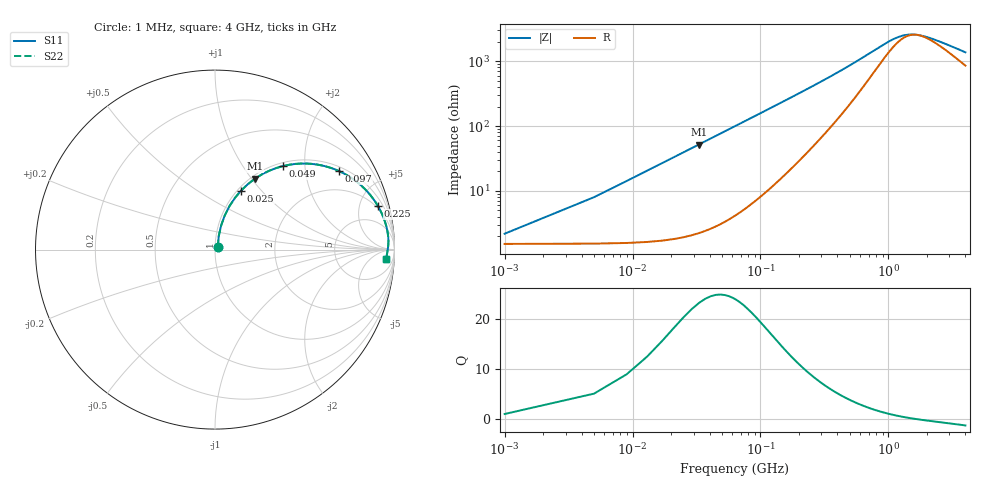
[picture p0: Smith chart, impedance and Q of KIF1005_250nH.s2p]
!version-2
!date-12.2020
!Series
# MHz S RI R 50
!Freq ReS11 ImS11 ReS21 ImS21 ReS12 ImS12 ReS22 ImS22
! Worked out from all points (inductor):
!   1001 points, 1 MHz to 4 GHz, reference 50 ohm
!   read as one part in series: L = 250 nH near 21 MHz
!   highest Q = 22.9 at 33 MHz (marker M1), where L = 250 nH
!   self-resonance near 1.67 GHz
!   S11 on the Smith chart (normalised r, x): 1 MHz: 1.03, +0.03; 25 MHz: 1.04, +0.79; 49 MHz: 1.06, +1.54; 97 MHz: 1.15, +3.06; 225 MHz: 1.73, +7.18; 4 GHz: 18, -21
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1  0.0152 0.0152  0.9848 -0.0152  0.9848 -0.0152  0.0152 0.0152
13  0.0542 0.1899  0.9458 -0.1899  0.9458 -0.1899  0.0542 0.1899
25  0.1457 0.3291  0.8543 -0.3291  0.8543 -0.3291  0.1457 0.3291
33  0.2218 0.3945  0.7782 -0.3945  0.7782 -0.3945  0.2218 0.3945
49  0.3773 0.4651  0.6227 -0.4651  0.6227 -0.4651  0.3773 0.4651
73  0.5662 0.4742  0.4338 -0.4742  0.4338 -0.4742  0.5662 0.4742
97  0.6917 0.4372  0.3083 -0.4372  0.3083 -0.4372  0.6917 0.4372
121  0.7721 0.3911  0.2279 -0.3911  0.2279 -0.3911  0.7721 0.3911
149  0.8315 0.3411  0.1685 -0.3411  0.1685 -0.3411  0.8315 0.3411
225  0.9074 0.2433  0.0926 -0.2433  0.0926 -0.2433  0.9074 0.2433
309  0.9385 0.1791  0.0615 -0.1791  0.0615 -0.1791  0.9385 0.1791
409  0.9539 0.1325  0.0461 -0.1325  0.0461 -0.1325  0.9539 0.1325
669  0.9651 0.0708  0.0349 -0.0708  0.0349 -0.0708  0.9651 0.0708
841  0.9662 0.0488  0.0338 -0.0488  0.0338 -0.0488  0.9662 0.0488
1009  0.9659 0.0338  0.0341 -0.0338  0.0341 -0.0338  0.9659 0.0338
1169  0.9652 0.0229  0.0348 -0.0229  0.0348 -0.0229  0.9652 0.0229
1337  0.9642 0.0137  0.0358 -0.0137  0.0358 -0.0137  0.9642 0.0137
1609  0.9626 0.00219  0.0374 -0.00219  0.0374 -0.00219  0.9626 0.00219
2001  0.9606 -0.0104  0.0394 0.0104  0.0394 0.0104  0.9606 -0.0104
2669  0.9578 -0.0267  0.0422 0.0267  0.0422 0.0267  0.9578 -0.0267
3337  0.9557 -0.0401  0.0443 0.0401  0.0443 0.0401  0.9557 -0.0401
4000  0.9538 -0.052  0.0462 0.052  0.0462 0.052  0.9538 -0.052
